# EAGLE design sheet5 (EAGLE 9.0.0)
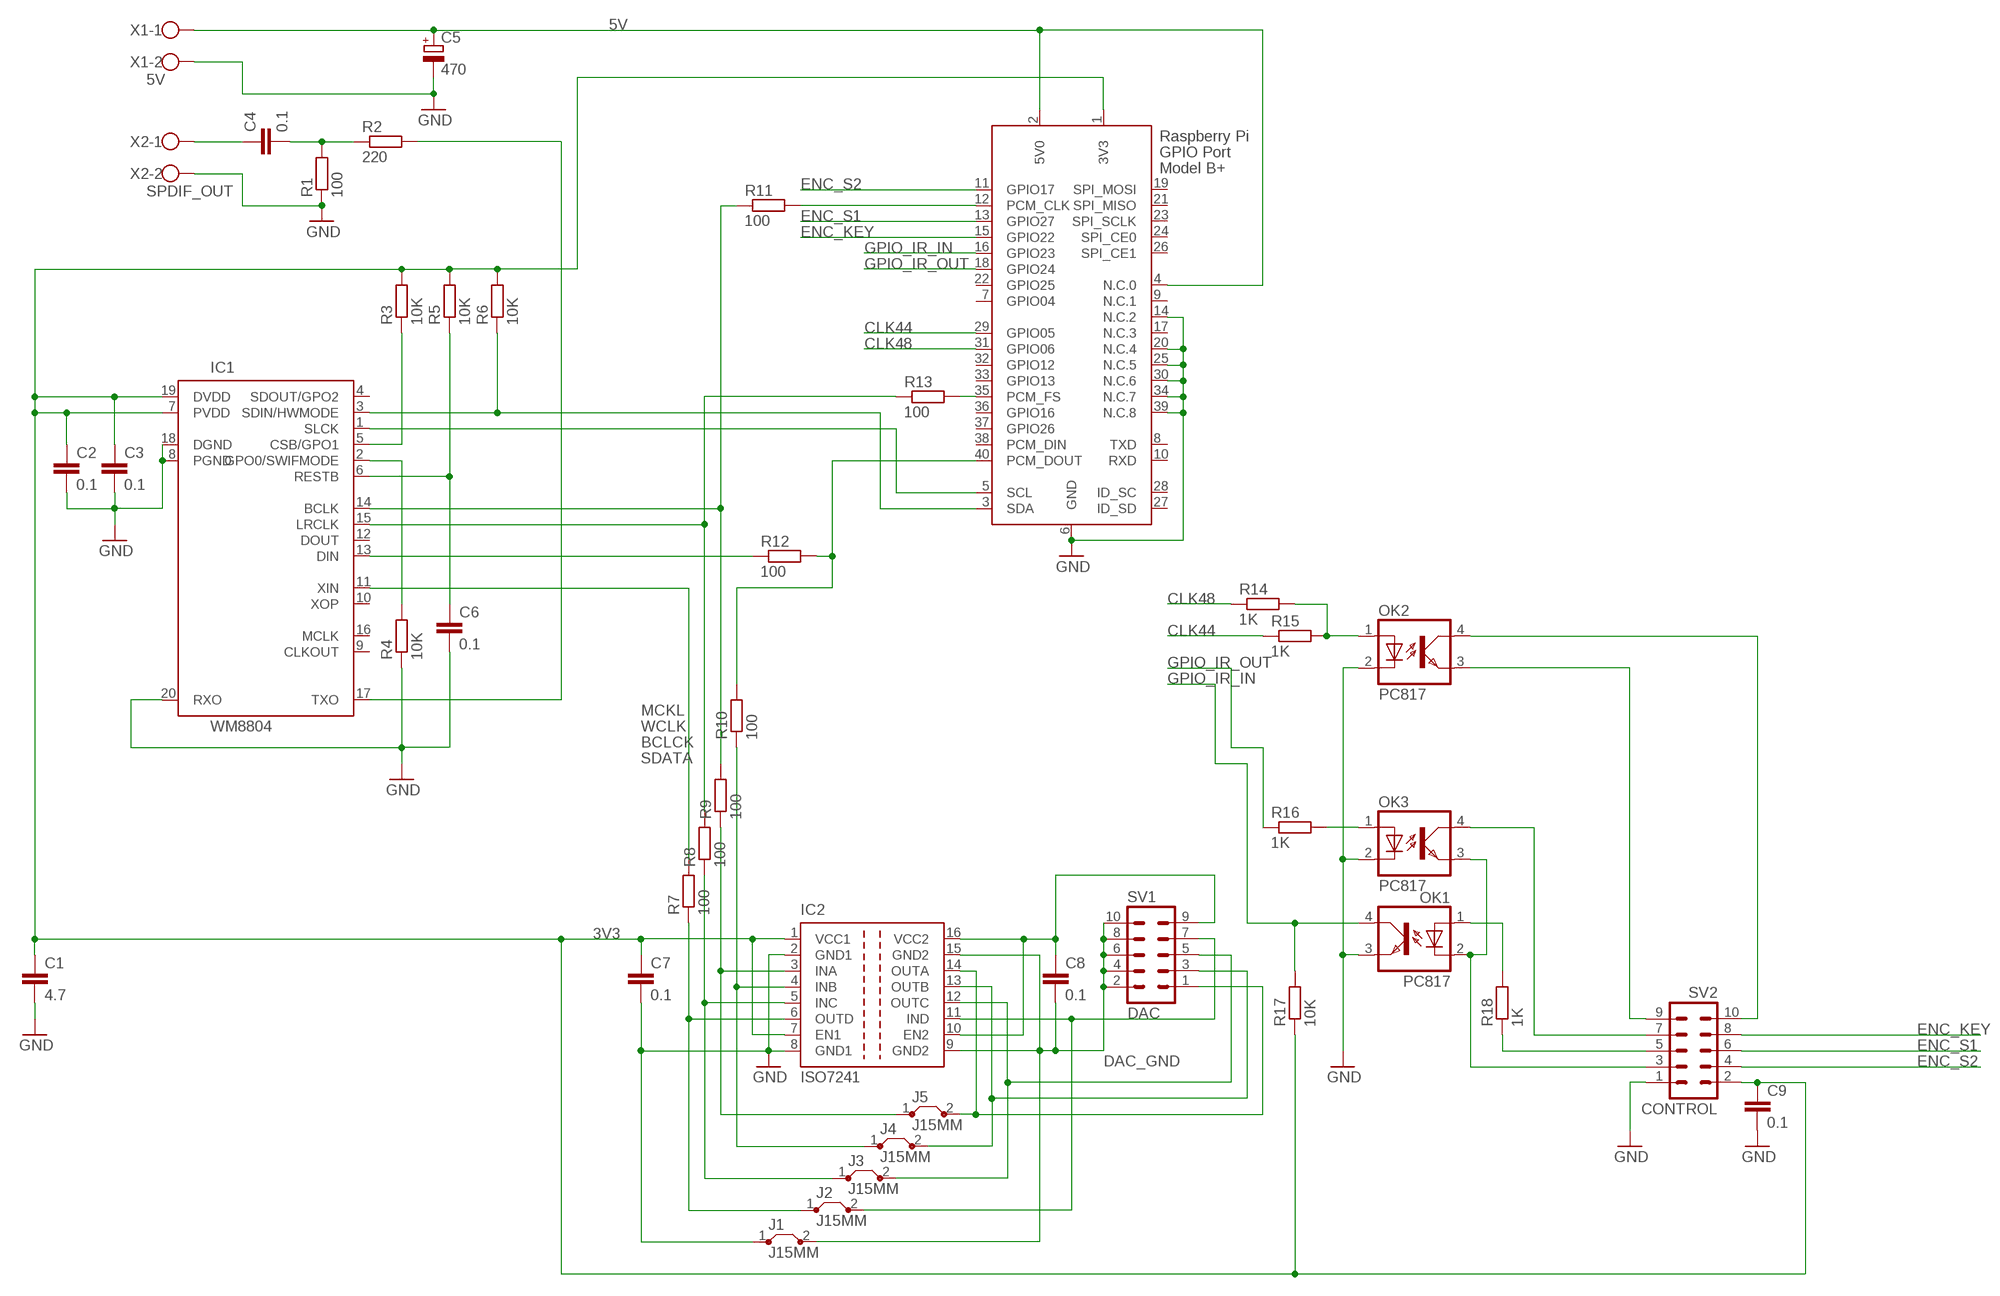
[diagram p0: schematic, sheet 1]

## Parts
C1  4.7  C-EU050-024X044  [C050-024X044]
C2  0.1  C-EUC1206  [C1206]
C3  0.1  C-EUC1206  [C1206]
C4  0.1  C-EU050-030X075  [C050-030X075]
C5  470  CPOL-EUE3.5-8  [E3,5-8]
C6  0.1  C-EUC1206  [C1206]
C7  0.1  C-EUC1206  [C1206]
C8  0.1  C-EUC1206  [C1206]
C9  0.1  C-EUC1206  [C1206]
IC1  WM8804  [SSOP20]
IC2  ISO7241  [SO-16DW]
J1  J15MM  [15]
J2  J15MM  [15]
J3  J15MM  [15]
J4  J15MM  [15]
J5  J15MM  [15]
OK1  PC817  [DIL04]
OK2  PC817  [DIL04]
OK3  PC817  [DIL04]
R1  100  R-EU_0207/10  [0207/10]
R2  220  R-EU_0207/10  [0207/10]
R3  10K  R-EU_R1206  [R1206]
R4  10K  R-EU_R1206  [R1206]
R5  10K  R-EU_R1206  [R1206]
R6  10K  R-EU_R1206  [R1206]
R7  100  R-EU_R1206  [R1206]
R8  100  R-EU_R1206  [R1206]
R9  100  R-EU_R1206  [R1206]
R10  100  R-EU_R1206  [R1206]
R11  100  R-EU_R1206  [R1206]
R12  100  R-EU_R1206  [R1206]
R13  100  R-EU_R1206  [R1206]
R14  1K  R-EU_R1206  [R1206]
R15  1K  R-EU_R1206  [R1206]
R16  1K  R-EU_R1206  [R1206]
R17  10K  R-EU_R1206  [R1206]
R18  1K  R-EU_R1206  [R1206]
SV1  DAC  ML10  [ML10]
SV2  CONTROL  ML10  [ML10]
X1  5V  W237-102  [W237-102]
X2  SPDIF_OUT  W237-102  [W237-102]
X3  RASPI_BOARD_B+_H  [RASPI_BOARD_B+HAT]

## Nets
3V3: C1.1 C2.1 C3.1 C7.1 C9.1 IC1.7(PVDD) IC1.19(DVDD) IC2.1(VCC1) IC2.7(EN1) R3.2 R5.2 R6.2 R17.1 SV2.2 X3.1(3V3)
5V: C5.+ X1.1 X3.2(5V0) X3.4(N.C.0)
$111: IC2.4(INB) J4.1 R10.1
BCLCK: IC2.3(INA) J5.1 R9.1
BCLK: IC1.14(BCLK) R9.2 R11.1
CLK44: R15.1 X3.29(GPIO05)
CLK48: R14.1 X3.31(GPIO06)
DAC_GND: C8.2 IC2.9(GND2) IC2.15(GND2) J1.2 SV1.2 SV1.4 SV1.6 SV1.8 SV1.10
ENC_KEY: SV2.8 X3.15(GPIO22)
ENC_S1: SV2.6 X3.13(GPIO27)
ENC_S2: SV2.4 X3.11(GPIO17)
GND [power]: C1.2 C2.2 C3.2 C5.- C6.2 C7.2 C9.2 IC1.8(PGND) IC1.18(DGND) IC1.20(RXO) IC2.2(GND1) IC2.8(GND1) J1.1 OK1.3(EMIT) OK2.2(C) OK3.2(C) R1.1 R4.1 SV2.1 X1.2 X2.2 X3.6(GND) X3.14(N.C.2) X3.20(N.C.4) X3.25(N.C.5) X3.30(N.C.6) X3.34(N.C.7) X3.39(N.C.8)
GPIO_IR_IN: OK1.4(COL) R17.2 X3.16(GPIO23)
GPIO_IR_OUT: R16.1 X3.18(GPIO24)
MCKL: IC1.11(XIN) R7.2
N$1: IC1.1(SLCK) X3.5(SCL)
N$2: IC1.3(SDIN/HWMODE) R6.1 X3.3(SDA)
N$3: C4.2 R1.2 R2.1
N$5: IC1.13(DIN) R12.1
N$6: IC1.17(TXO) R2.2
N$7: R11.2 X3.12(PCM_CLK)
N$8: R13.2 X3.35(PCM_FS)
N$9: C4.1 X2.1
N$10: IC2.6(OUTD) J2.1 R7.1
N$11 [power]: IC1.2(GPO0/SWIFMODE) R4.2
N$13: IC2.5(INC) J3.1 R8.1
N$15: OK2.1(A) R14.2 R15.2
N$16: IC1.5(CSB/GPO1) R3.1
N$18: OK1.2(C) OK3.3(EMIT) SV2.3
N$19: C6.1 IC1.6(RESTB) R5.1
N$21: R18.1 SV2.5
N$22: OK2.3(EMIT) SV2.9
N$23: IC2.11(IND) J2.2 SV1.7
N$24: C8.1 IC2.10(EN2) IC2.16(VCC2) SV1.9
N$25: OK3.4(COL) SV2.7
N$26: OK3.1(A) R16.2
N$27: OK1.1(A) R18.2
N$28: OK2.4(COL) SV2.10
N$29: IC2.12(OUTC) J3.2 SV1.5
N$31: IC2.13(OUTB) J4.2 SV1.3
N$32: IC2.14(OUTA) J5.2 SV1.1
SDATA: R10.2 R12.2 X3.40(PCM_DOUT)
WCLK: IC1.15(LRCLK) R8.2 R13.1
Unconnected: IC1.4(SDOUT/GPO2) IC1.9(CLKOUT) IC1.10(XOP) IC1.12(DOUT) IC1.16(MCLK) X3.7(GPIO04) X3.8(TXD) X3.9(N.C.1) X3.10(RXD) X3.17(N.C.3) X3.19(SPI_MOSI) X3.21(SPI_MISO) X3.22(GPIO25) X3.23(SPI_SCLK) X3.24(SPI_CE0) X3.26(SPI_CE1) X3.27(ID_SD) X3.28(ID_SC) X3.32(GPIO12) X3.33(GPIO13) X3.36(GPIO16) X3.37(GPIO26) X3.38(PCM_DIN)

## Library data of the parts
C1-C4 C6-C9 = rcl:C-EU: CAPACITOR, European symbol; SPICEPREFIX: C
C5 = rcl:CPOL-EU: POLARIZED CAPACITOR, European symbol; SPICEPREFIX: C
IC1 = wm8804:WM8804: TRANSCEIVER, S/PDIF, 1:1, 20SSOP Supply Voltage Range: 2.7V to 3.6V Logic Case Style: SSOP No. of Pins: 20 Operating Temperature Range: -40°C to +85°C SVHC: No SVHC (19-Dec-2011) Interface Type: Serial, 2 / 3 Wire Line / Bus Driver / Receiver / Transceiver Type: Digital Interface Transceiver with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
IC2 = texas:ISO7241: HIGH SPEED QUAD DIGITAL ISOLATORS Source: http://focus.ti.com/lit/ds/symlink/iso7240m.pdf; MPN: ISO7241CDW; OC_FARNELL: 1575372; OC_NEWARK: 73M3155
J1-J5 = jumper:J: Bridge
OK1-OK3 = optocoupler:PC817: SHARP OPTO COUPLER; MPN: PC817X4J000F; OC_FARNELL: 9707727; OC_NEWARK: 97K7059
R1-R18 = rcl:R-EU_: RESISTOR, European symbol; SPICEPREFIX: R
SV1 SV2 = con-ml:ML10: HARTING; OC_FARNELL: unknown; OC_NEWARK: unknown
X1 X2 = con-wago-500:W237-102: WAGO SCREW CLAMP; MPN: 237-102; OC_FARNELL: unknown; OC_NEWARK: 70K9898
X3 = raspberrypi_bastelstube_v13:RASPI_BOARD_B+: Raspberry Pi GPIO connector with markings for the outer dimensions of the Raspberry Pi board model B+ with different sets of drill holes or mounting pads

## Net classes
0 default: width 0.254 mm, drill 0.254 mm, clearance 0.254 mm
1 power: width 0.305 mm, drill 0.305 mm, clearance 0.305 mm

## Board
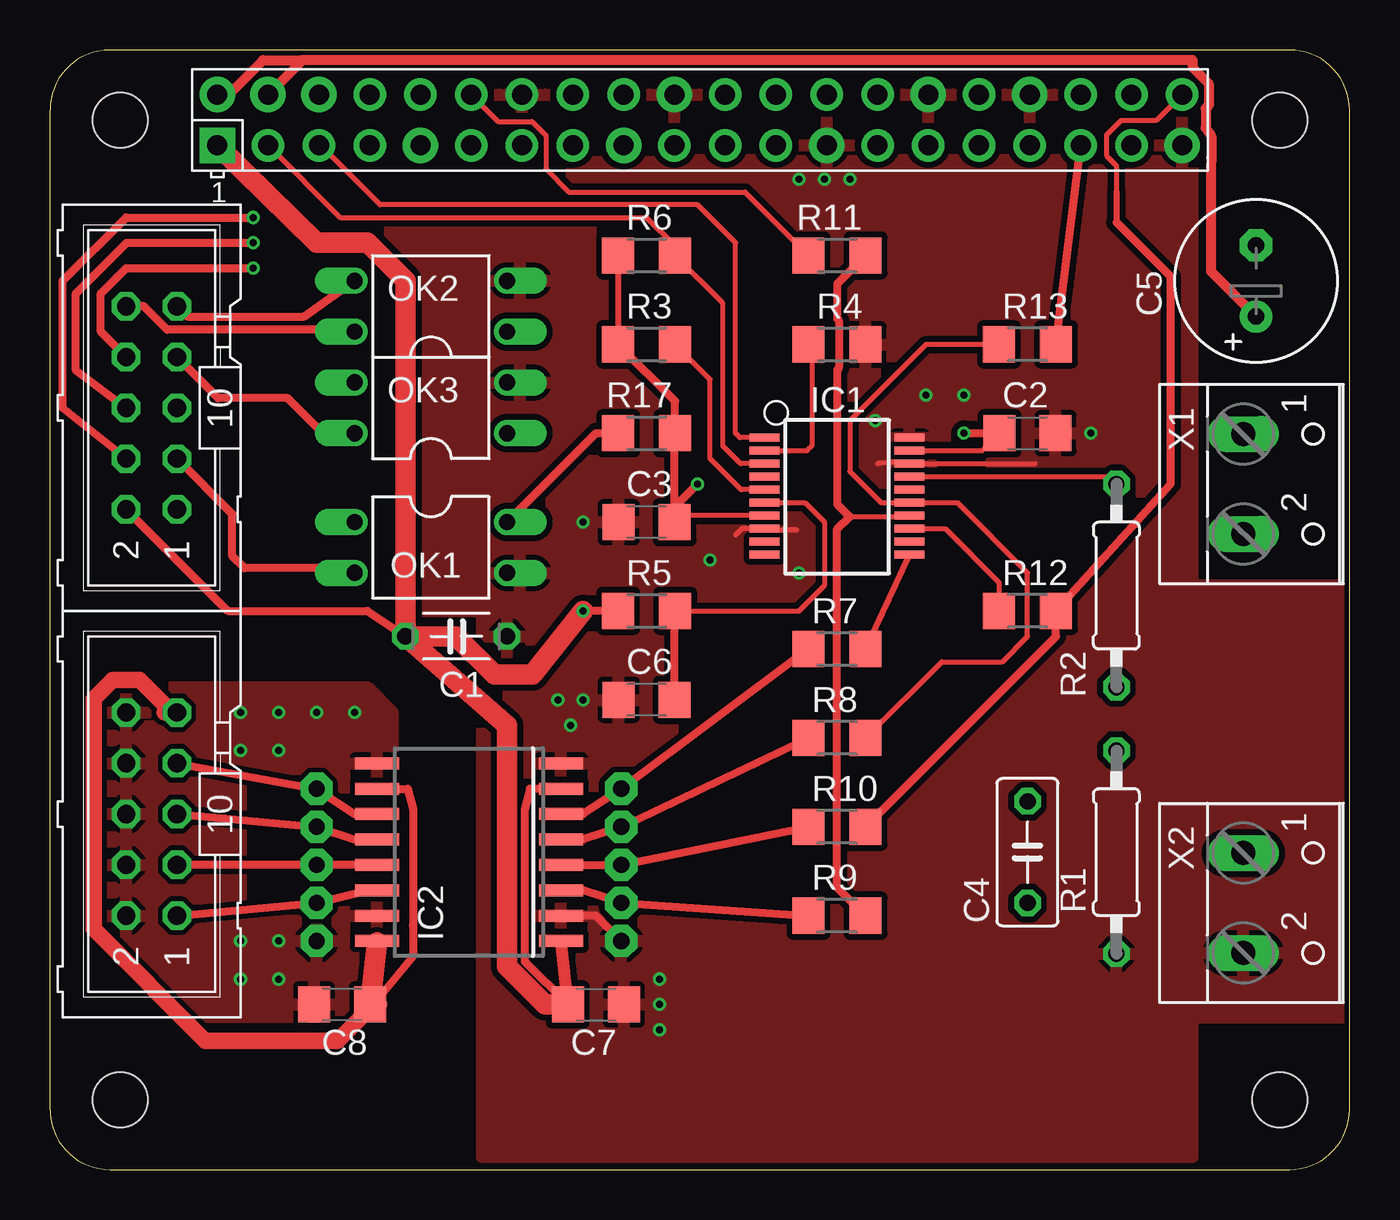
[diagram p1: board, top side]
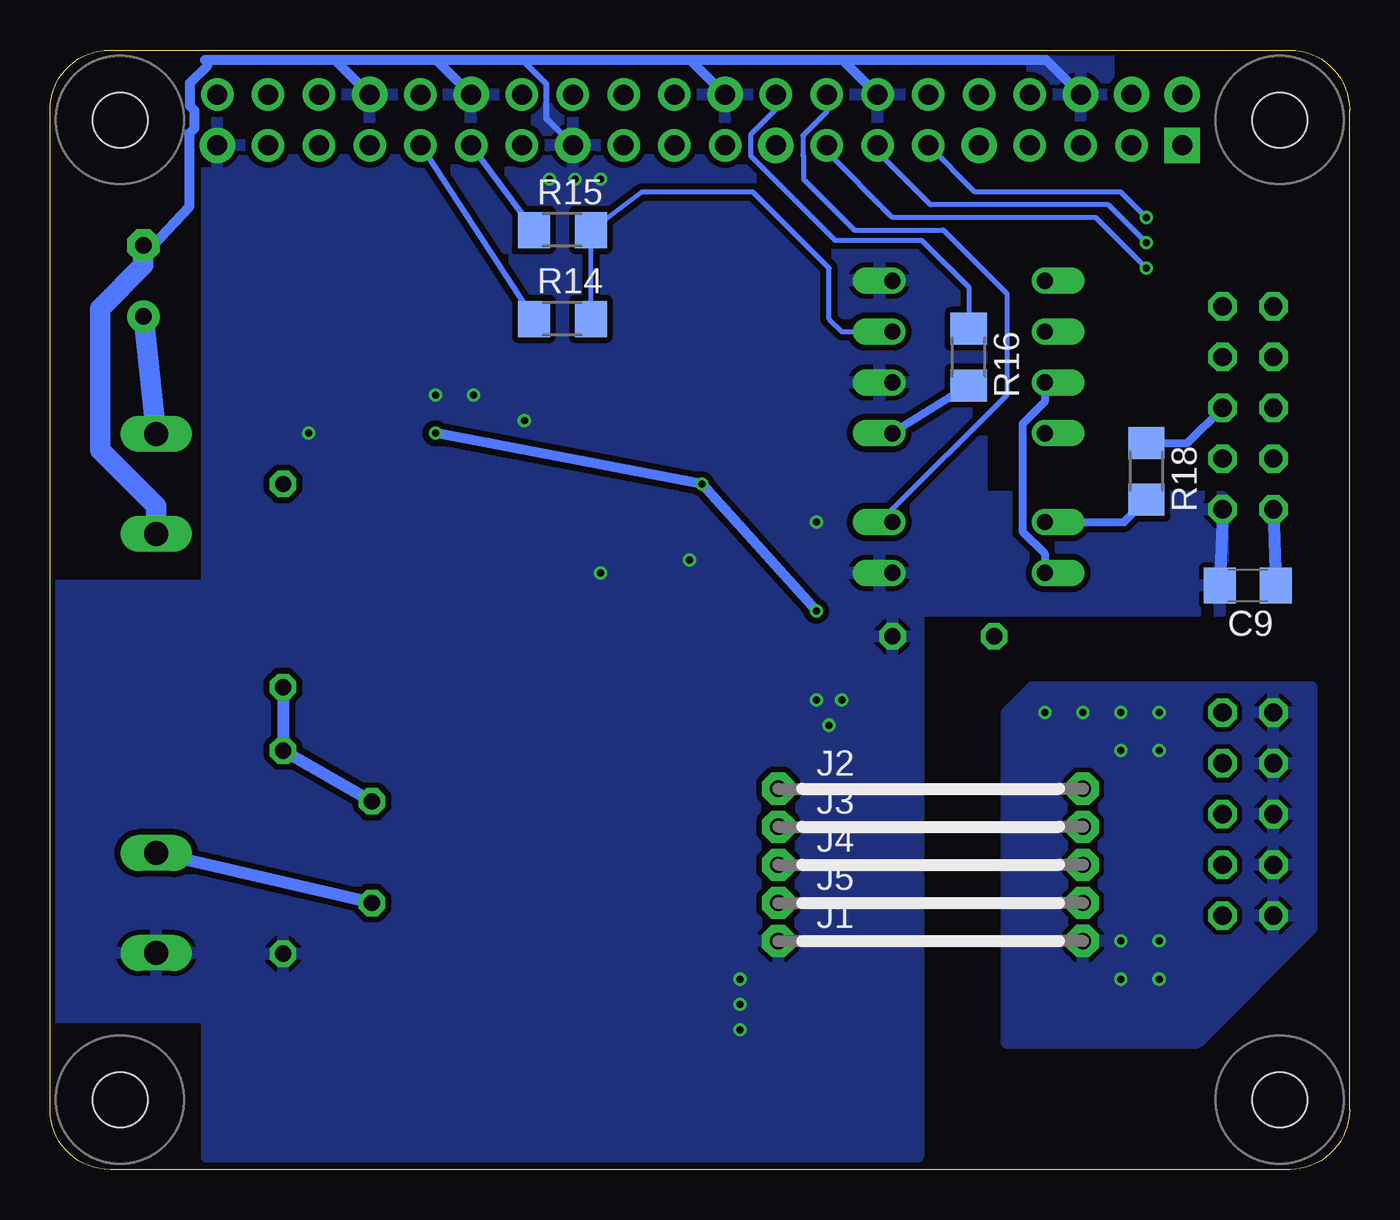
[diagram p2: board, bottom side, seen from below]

Size 65 x 56 mm. Coordinates in mm from the lower left corner, seen from the top.
Copper layers (1*16): Top 0.035mm / dielectric 1.5mm / Bottom 0.035mm
Design rules "SeeedStudio_2layer_DRU_no_angle_20140221": minimum track width 6mil, minimum drill 12mil, track to track 6mil, track to pad 6mil, pad to pad 6mil, via to via 6mil, smd to smd 0mil, copper to edge 10mil, drill to drill 10mil, minimum pad ring 10mil, minimum via ring 6mil, stop-mask expansion 2mil, vias tented up to drill 100mil, thermal gap 10mil

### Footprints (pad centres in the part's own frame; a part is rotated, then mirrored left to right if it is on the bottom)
C050-024X044 = drill 0.813 octagon: 1 -2.54,0; 2 2.54,0
C1206 = smd 1.6 x 1.8: 1 -1.4,0; 2 1.4,0
C050-030X075 = drill 0.813 octagon: 1 -2.54,0; 2 2.54,0
E3,5-8 = drill 0.813 pad 1.6: + -1.778,0 | drill 0.813 pad 1.6 octagon: - 1.778,0
SSOP20 = smd 0.4 x 1.5: 1 -2.955,-3.625; 2 -2.305,-3.625; 3 -1.655,-3.625; 4 -1.005,-3.625; 5 -0.355,-3.625; 6 0.295,-3.625; 7 0.945,-3.625; 8 1.595,-3.625; 9 2.245,-3.625; 10 2.895,-3.625; 11 2.895,3.625; 12 2.245,3.625; 13 1.595,3.625; 14 0.945,3.625; 15 0.295,3.625; 16 -0.355,3.625; 17 -1.005,3.625; 18 -1.655,3.625; 19 -2.305,3.625; 20 -2.955,3.625
SO-16DW = smd 0.6 x 2.2: 1 -4.445,-4.6; 2 -3.175,-4.6; 3 -1.905,-4.6; 4 -0.635,-4.6; 5 0.635,-4.6; 6 1.905,-4.6; 7 3.175,-4.6; 8 4.445,-4.6; 9 4.445,4.6; 10 3.175,4.6; 11 1.905,4.6; 12 0.635,4.6; 13 -0.635,4.6; 14 -1.905,4.6; 15 -3.175,4.6; 16 -4.445,4.6
15 = drill 0.813 pad 1.6 octagon: 1 -7.62,0; 2 7.62,0
DIL04 = drill 0.813 offset: 1 -1.27,-3.81; 2 1.27,-3.81; 3 1.27,3.81; 4 -1.27,3.81
0207/10 = drill 0.813 octagon: 1 -5.08,0; 2 5.08,0
R1206 = smd 1.6 x 1.803: 1 -1.422,0; 2 1.422,0
ML10 = drill 0.914 octagon: 1 -5.08,-1.27; 2 -5.08,1.27; 3 -2.54,-1.27; 4 -2.54,1.27; 5 0,-1.27; 6 0,1.27; 7 2.54,-1.27; 8 2.54,1.27; 9 5.08,-1.27; 10 5.08,1.27
W237-102 = drill 1.194 long: 1 -2.5,-1.27; 2 2.5,-1.27
RASPI_BOARD_B+HAT = drill 1 pad 1.778 square: 1 8.37,51.23 | drill 1 pad 1.778: 2 8.37,53.77; 4 10.91,53.77; 6 13.45,53.77; 9 18.53,51.23; 17 28.69,51.23; 20 31.23,53.77; 25 38.85,51.23; 30 43.93,53.77; 34 49.01,53.77; 39 56.63,51.23 | drill 1 pad 1.626: 3 10.91,51.23; 5 13.45,51.23; 7 15.99,51.23; 8 15.99,53.77; 10 18.53,53.77; 11 21.07,51.23; 12 21.07,53.77; 13 23.61,51.23; 14 23.61,53.77; 15 26.15,51.23; 16 26.15,53.77; 18 28.69,53.77; 19 31.23,51.23; 21 33.77,51.23; 22 33.77,53.77; 23 36.31,51.23; 24 36.31,53.77; 26 38.85,53.77; 27 41.39,51.23; 28 41.39,53.77; 29 43.93,51.23; 31 46.47,51.23; 32 46.47,53.77; 33 49.01,51.23; 35 51.55,51.23; 36 51.55,53.77; 37 54.09,51.23; 38 54.09,53.77; 40 56.63,53.77 | hole 2.75: 3.5,3.5; 3.5,52.5; 61.5,3.5; 61.5,52.5

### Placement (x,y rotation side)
C1  20.32,26.67 0 top
C2  48.9,36.83 0 top
C3  29.84,32.38 180 top
C4  48.9,15.88 90 top
C5  60.33,44.45 90 top
C6  29.84,23.5 180 top
C7  27.3,8.26 0 top
C8  14.61,8.26 180 top
C9  5.08,29.21 180 bottom
IC1  39.37,33.66 270 top
IC2  20.95,15.88 90 top
J1  20.95,11.43 0 bottom
J2  20.95,19.05 0 bottom
J3  20.95,17.14 0 bottom
J4  20.95,15.24 0 bottom
J5  20.95,13.34 0 bottom
OK1  19.05,31.11 270 top
OK2  19.05,43.18 90 top
OK3  19.05,38.1 90 top
R1  53.34,15.88 90 top
R2  53.34,29.21 90 top
R3  29.84,41.27 180 top
R4  39.37,41.27 180 top
R5  29.84,27.94 180 top
R6  29.84,45.72 180 top
R7  39.37,26.04 0 top
R8  39.37,21.59 0 top
R9  39.37,12.7 0 top
R10  39.37,17.14 0 top
R11  39.37,45.72 180 top
R12  48.9,27.94 0 top
R13  48.9,41.27 0 top
R14  39.37,42.55 0 bottom
R15  39.37,46.99 0 bottom
R16  19.05,40.64 270 bottom
R17  29.84,36.83 180 top
R18  10.16,34.92 270 bottom
SV1  5.08,17.78 90 top
SV2  5.08,38.1 90 top
X1  60.96,34.29 270 top
X2  60.96,13.34 270 top
X3  0,0 0 top

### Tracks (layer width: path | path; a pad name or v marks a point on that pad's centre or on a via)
3V3  (via drill 0.35)
  Top 0.254: IC1.7 31.57,32.71 C3.1 | IC1.19 46.62,35.96 C2.1
  Top 0.305: R6.2 R3.2
  Top 0.406: IC2.7 24.79,19.05 24.01,19.05 23.74,18.02 23.74,12.11 23.75,12.1 23.75,10.41 C7.1 | SV2.2 8.89,27.94 15.88,27.94 C1.1 | 31.25,32.64 31.25,33.02 C3.1 | v45.72,36.83 C2.1 | 31.25,33.15 31.25,36.81 R17.1 31.27,38.43 R3.2 | C3.1 | C3.1 31.25,33.15 | 31.25,33.15 v32.38,34.29 | R5.2 v26.67,27.94
  Top 0.61: C7.1 IC2.1
  Top 1.016: C7.1 24.77,8.26 22.86,10.16 22.86,22.23 C1.1 | SV2.2 3.91,33.02 | X3.1 13.34,46.35 15.88,46.35 17.78,44.45 C1.1 | C1.1 20.32,26.67 22.23,24.77 24.13,24.77 v26.67,27.94
  Bottom 0.508: v26.67,27.94 v32.38,34.29 v45.72,36.83
  Bottom 0.61: SV2.2 C9.1
5V
  Top 0.508: X3.2 8.93,53.77 10.66,55.49 12.63,55.49 | 12.63,55.49 57.15,55.49 57.15,55.12 57.95,54.32 57.95,53.22 57.81,53.08 57.81,52.1 58.08,51.7 58.08,50.63 58.06,50.11 58.06,44.93 C5.+ | X3.4 12.63,55.49
  Bottom 1.016: X1.1 60.24,41.92 C5.+
$111
  Top 0.406: IC2.4 J4.1 R10.1
BCLCK
  Top 0.406: IC2.3 26.67,13.97 J5.1 R9.1
BCLK
  Top 0.254: 39.98,32.67 40.01,32.67 42.95,32.67
  Top 0.305: 43.04,32.67 IC1.14 42.95,32.67
  Top 0.406: 39.98,32.67 39.37,33.28 39.37,39.99 39.46,40.08 39.46,42.47 39.37,42.56 39.37,44.3 R11.1 | R9.2 39.37,14.12 39.37,32.03 40.01,32.67
CLK44
  Bottom 0.305: R15.1 X3.29
CLK48
  Bottom 0.305: X3.31 R14.1
DAC_GND  (via drill 0.35)
  Top 0.406: 16.04,12.7 IC2.15
  other vias: 9.53,20.95 11.43,20.95 11.43,11.43 9.53,11.43 9.53,22.86 11.43,22.86 13.34,22.86 9.53,9.53 11.43,9.53 15.24,22.86
  pour Top: 2.54,24.13 15.88,24.13 17.14,22.86 17.14,19.05 9.53,19.05 9.53,13.34 17.14,13.34 17.14,7.62 2.54,7.62
  pour Bottom: 15.88,24.13 1.91,24.13 1.91,12.06 7.62,6.35 17.14,6.35 17.14,22.86
ENC_KEY  (via drill 0.35)
  Top 0.406: SV2.8 2.54,41.91 2.54,43.81 3.81,45.09 v10.16,45.09
  Bottom 0.254: v10.16,45.09 12.7,47.62 22.86,47.62 26.15,50.91 X3.15
ENC_S1  (via drill 0.35)
  Top 0.406: SV2.6 1.29,39.98 1.29,43.81 3.83,46.35 v10.16,46.35
  Bottom 0.254: v10.16,46.35 12.06,48.26 20.95,48.26 23.61,50.91 X3.13
ENC_S2  (via drill 0.35)
  Top 0.406: SV2.4 0.64,38.1 0.64,44.45 3.81,47.62 v10.16,47.62
  Bottom 0.254: v10.16,47.62 11.43,48.9 18.73,48.9 X3.11
GND  (via drill 0.35)
  Top 0.254: 34.29,31.75 34.6,32.06 IC1.8 35.81,31.99 36.65,31.99 36.77,32 37.34,32 | 49.28,35.31 IC1.18 42.93,35.38 42.09,35.38 41.4,35.31
  Top 0.406: J1.1 27.3,12.7 IC2.2
  Bottom 0.305: X3.25 40.17,52.55 40.17,54.27 41.27,55.38 41.27,55.49
  Bottom 0.508: 25.33,55.49 15.17,55.49 X3.6 13.24,53.77 | 25.33,55.49 32.95,55.49 | 32.95,55.49 41.27,55.49 45.65,55.49 | 45.65,55.49 50.73,55.49 | 50.73,55.49 57.15,55.49 | 57.15,55.49 57.24,55.49 | X3.14 25.33,55.49 | X3.20 32.95,55.49 | X3.30 45.65,55.49 | X3.34 50.73,55.49 | 57.15,55.49 57.15,55.19 58,54.34 58,53.2 57.78,52.98 57.78,52.07 58.04,51.82 58.04,48.13 59.82,46.23 C5.-
  Bottom 0.61: SV2.1 C9.2
  Bottom 1.016: X1.2 59.69,33.19 62.5,36 62.5,43.07 60.33,45.24 C5.-
  other vias: 26.67,23.5 26.04,22.23 25.4,23.5 40.01,49.53 38.73,49.53 41.27,37.47 37.47,29.84 33.02,30.48 30.48,8.26 37.47,49.53 26.67,32.38 52.07,36.83 30.48,9.53 30.48,6.99 43.81,38.73 45.72,38.73
  pour Bottom: 57.15,0.64 57.15,7.62 64.77,7.62 64.77,29.21 57.15,29.21 57.15,53.98 15.88,53.98 15.88,55.88 12.06,55.88 12.06,52.7 18.41,52.7 18.41,33.66 6.35,33.66 6.35,27.94 21.59,27.94 21.59,0.64
  pour Top: 57.15,53.98 20.32,53.98 20.32,49.53 12.06,49.53 12.06,27.94 21.59,27.94 21.59,0.64 57.15,0.64 57.15,7.62 64.77,7.62 64.77,29.21 57.15,29.21
GPIO_IR_IN
  Top 0.254: OK1.4 24.54,32.38
  Top 0.406: OK1.4 27.3,36.83 R17.2
  Bottom 0.254: X3.16 26.15,52.92 27.34,51.72 27.34,50.74 27.3,50.7 27.3,49.53 24.77,46.99 20.32,46.99 17.14,43.81 17.14,38.73 23.18,32.7 | 23.18,32.7 23.5,32.38 | OK1.4 23.18,32.7
GPIO_IR_OUT
  Bottom 0.254: R16.1 19.05,44.13 21.4,46.48 25.74,46.48 29.96,50.7 29.96,51.76 28.69,53.03 X3.18
MCKL
  Top 0.305: R7.2 IC1.11
N$1
  Top 0.254: X3.5 13.54,51.23 16.51,48.26 32.38,48.26 34.29,46.35 34.29,36.83 34.51,36.61 IC1.1
N$2
  Top 0.254: X3.3 14.52,47.62 29.84,47.62 31.27,46.2 R6.1 33.66,43.33 33.66,36.2 34.54,35.31 IC1.3
  Top 0.406: X3.3
N$3
  Bottom 0.61: R2.1 R1.2 C4.2
N$5
  Top 0.254: IC1.13 44.77,32.06 47.47,29.36 R12.1
  Top 0.305: IC1.13 43.04,32.02
N$6
  Top 0.254: IC1.17 52.97,34.66 R2.2
N$7
  Top 0.254: X3.12 22.42,52.42 24.1,52.42 24.8,51.72 24.8,50.04 25.95,48.9 34.77,48.9 R11.2
N$8
  Top 0.406: R13.2 X3.35
N$9
  Bottom 0.61: C4.1 X2.1
N$10
  Top 0.406: IC2.6 26.67,17.78 J2.1 R7.1
N$11
  Top 0.254: IC1.2 37.87,35.96 38.1,36.2 38.1,41.12 R4.2
N$13
  Top 0.406: IC2.5 26.67,16.51 J3.1 R8.1
N$15
  Bottom 0.254: OK2.1 25.4,41.91 26.04,42.55 26.04,45.09 29.84,48.9 35.41,48.9 R15.2 R14.2
N$16
  Top 0.254: IC1.5 34.57,34.01 33.02,35.56 33.02,39.52 R3.1
N$18
  Top 0.406: OK1.2 15.01,30.08 9.73,30.08 9.12,30.68 9.12,32.79 SV2.3
  Bottom 0.406: OK3.3 15.24,38.41 16.36,37.29 16.36,31.92 15.24,30.8 OK1.2 | SV2.3 6.35,35.03
N$19
  Top 0.254: IC1.6 37.76,33.36 38.73,32.38 38.73,29.21 37.44,27.92 31.25,27.92
  Top 0.305: 35.7,33.32 IC1.6
  Top 0.406: C6.1 31.25,27.92 R5.1
N$21
  Bottom 0.406: R18.1 8.1,36.35 SV2.5
N$22
  Top 0.406: SV2.9 6.86,42.67 12.7,42.67 OK2.3
  Bottom 0.406: OK2.3 13.97,44.45
N$23
  Top 0.406: IC2.11 15.24,17.78 J2.2 SV1.7
N$24
  Top 0.406: IC2.10 16.74,19.05 17.9,19.05 18.17,18.02 18.17,12.21 18.16,12.21 18.16,10.67 16.04,8.09
  Top 0.813: 5.75,22.86 SV1.9 6.11,22.86 4.48,24.49 3.14,24.49 2.18,23.53 2.18,12.03 7.77,6.44 14.38,6.44 16.04,8.09 16.2,8.26 | 16.2,8.26 C8.1 | 16.36,11.36 IC2.16 | 16.47,8.26 16.2,8.26
  Top 1.016: C8.1 16.36,11.36
N$25
  Top 0.406: OK3.4 13.65,36.83 11.89,38.58 8.41,38.58 SV2.7
N$26
  Bottom 0.406: R16.2 OK3.1
N$27
  Bottom 0.406: OK1.1 11.28,32.38 R18.2
N$28
  Top 0.406: SV2.10 4.7,43.18 5.87,42.01 15.14,42.01 OK2.4
N$29
  Top 0.406: IC2.12 15.24,16.51 J3.2 SV1.5
N$31
  Top 0.406: IC2.13 J4.2 SV1.3
N$32
  Top 0.406: IC2.14 15.88,13.97 J5.2 SV1.1
SDATA
  Top 0.254: X3.40 55.34,52.48 53.57,52.48 52.84,51.75 52.84,50.71 53.34,50.22 53.34,48.9
  Top 0.305: 53.34,48.9 53.34,47.38
  Top 0.406: 53.34,47.38 56.06,44.66 56.06,34.29 R12.2 50.32,26.67 R10.2
WCLK
  Top 0.254: R13.1 43.81,41.27 40.01,37.47 40.01,34.92 41.57,33.36 IC1.15 45.38,33.36 48.9,29.84 48.9,26.67 47.62,25.4 44.6,25.4 R8.2
  Top 0.305: 43.04,33.4 IC1.15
